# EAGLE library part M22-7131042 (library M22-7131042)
2.00mm (0.079") Pitch SIL Vertical 2.6mm Throughboard Socket Assembly, selective gold + tin, 10 contacts Source: Datasheet
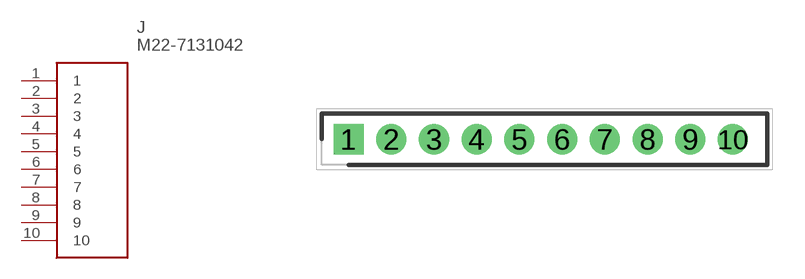
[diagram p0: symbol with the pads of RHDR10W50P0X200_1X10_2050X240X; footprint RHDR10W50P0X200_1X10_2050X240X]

Designator prefix J

## M22-7131042 (Description: 2.00mm (0.079") Pitch SIL Vertical 2.6mm Throughboard Socket Assembly, selective gold + tin, 10 contacts; Height: 4.4mm; Manufacturer_Name: Harwin; Manufacturer_Part_Number: M22-7131042; Mouser_Part_Number: 855-M22-7131042; Mouser_Price-Stock: https://www.mouser.co.uk/ProductDetail/Harwin/M22-7131042?qs=WS5Jv%252B%252Bx1qUfXs5lYp1U1g%3D%3D)  [RHDR10W50P0X200_1X10_2050X240X]
1  1
2  2
3  3
4  4
5  5
6  6
7  7
8  8
9  9
10  10

## Footprint RHDR10W50P0X200_1X10_2050X240X (pad centres in mm)
M22-7131042
drill 0.9 pad 1.35 square: 1 0,0
drill 0.9 pad 1.35: 2 2,0; 3 4,0; 4 6,0; 5 8,0; 6 10,0; 7 12,0; 8 14,0; 9 16,0; 10 18,0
